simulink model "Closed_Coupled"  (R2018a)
settings: Solver=ode45  StartTime=0.0  StopTime=60  RelTol=1e-3  EnableMultiTasking=on
InitFcn:
  | init
StartFcn:
  | init
StopFcn:
  | pl
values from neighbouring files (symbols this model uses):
  Aact = [0, 1; -omg^2, -2*zet*omg]    [init.m]
  Bact = [0; omg^2]    [init.m]
  Cact = [1, 0]    [init.m]
  Cyb = -0.0245    [init.m]    (also in lqr_des.m)
  Cydel = [-0.24668,0.24668, 0.47413,-0.47413,0]/100    [init.m]    (also in lqr_des.m = [-0.24668,0.24668, 0.47413,-0.47413]/100)
  Cza = -0.073    [init.m]
  Czdel = [0.51664,0.51664,0.60478,0.60478,0.06]/100    [init.m]
  d2r = pi/180    (= 0.0174532925199)    [init.m]
  Dact = 0    [init.m]
  Mass = 198.32    [init.m]    (also in lqr_des.m)
  Qbar = 150    [init.m]    (also in lqr_des.m)
  r2d = 180/pi    (= 57.2957795131)    [init.m]    (also in pl.m)
  Sref = 79.069    [init.m]    (also in lqr_des.m)
  V0 = 822.8    [init.m]
undefined symbols (not defined in the file or in its folder): Ap, Bp, Cp, Dp, K4axmix, Kpr, Kq

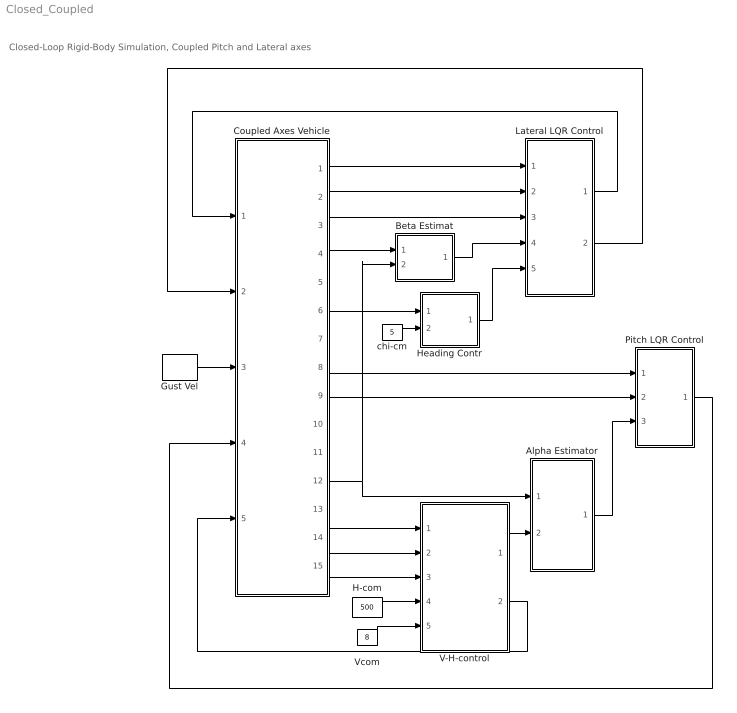
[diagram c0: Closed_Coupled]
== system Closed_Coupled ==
  note: Closed-Loop Rigid-Body Simulation, Coupled Pitch and Lateral axes
  Alpha Estimator : Subsystem
  Beta Estimat : Subsystem
  Coupled Axes Vehicle : Subsystem
  Gust Vel : DiscretePulseGenerator  PulseType=Time based  Amplitude=40  Period=100  PulseWidth=10  PhaseDelay=20
  H-com : Constant  Value=500
  Heading Contr : Subsystem
  Lateral LQR Control : Subsystem
  Pitch LQR Control : Subsystem
  V-H-control : Subsystem
  Vcom : Constant  Value=8
  chi-cm : Constant  Value=5
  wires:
  Coupled Axes Vehicle/2(p) -> Lateral LQR Control/2(p)
  Coupled Axes Vehicle/3(r) -> Lateral LQR Control/3(r)
  Coupled Axes Vehicle/1(phi) -> Lateral LQR Control/1(phi)
  Coupled Axes Vehicle/9(q) -> Pitch LQR Control/2(q)
  Coupled Axes Vehicle/8(thet) -> Pitch LQR Control/1(thet)
  Pitch LQR Control/1(elev) -> Coupled Axes Vehicle/4(pitch)
  Coupled Axes Vehicle/12(delt) -> Alpha Estimator/1(delta), Beta Estimat/2(delta)
  H-com/1 -> V-H-control/4(H-comd)
  Vcom/1 -> V-H-control/5(Vcomd)
  Alpha Estimator/1(alphat) -> Pitch LQR Control/3(alfa)
  V-H-control/1(Zdd-com) -> Alpha Estimator/2(Zdd)
  V-H-control/2(Throtle) -> Coupled Axes Vehicle/5(Ax-cmd)
  Lateral LQR Control/1(Ailer) -> Coupled Axes Vehicle/1(roll)
  Lateral LQR Control/2(Rud) -> Coupled Axes Vehicle/2(yaw)
  Coupled Axes Vehicle/4(Ny) -> Beta Estimat/1(Ydd)
  Beta Estimat/1(bethat) -> Lateral LQR Control/4(bet)
  chi-cm/1 -> Heading Contr/2(chi-cmd)
  Heading Contr/1(phi-cmd) -> Lateral LQR Control/5(ph-cmd)
  Coupled Axes Vehicle/6("chi ") -> Heading Contr/1(chi)
  Coupled Axes Vehicle/14(Nz) -> V-H-control/2(Az)
  Coupled Axes Vehicle/15(dH) -> V-H-control/3(dH)
  Coupled Axes Vehicle/13(V-dot) -> V-H-control/1(Vdot)
  Gust Vel/1 -> Coupled Axes Vehicle/3(Gust)

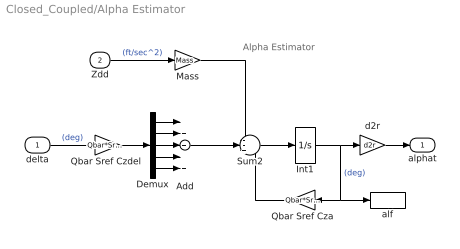
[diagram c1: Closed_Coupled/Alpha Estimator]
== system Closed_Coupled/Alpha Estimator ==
  note: Alpha Estimator
  delta : Inport
  Zdd : Inport  Port=2
  Add : Sum  Inputs=+++++
  Demux : Demux  Outputs=5
  Int1 : Integrator
  Mass : Gain  Gain=Mass
  Qbar Sref Cza : Gain  Gain=Qbar*Sref*Cza
  "Qbar Sref Czdel " : Gain  Gain=Qbar*Sref*Czdel
  Sum2 : Sum  Inputs=--+
  alf : ToWorkspace  VariableName=alphat  SampleTime=-1
  d2r : Gain  Gain=d2r
  alphat : Outport
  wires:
  Demux/5 -> Add/5
  Demux/4 -> Add/4
  Demux/3 -> Add/3
  Demux/2 -> Add/2
  Demux/1 -> Add/1
  "Qbar Sref Czdel "/1 -> Demux/1
  delta/1 -> "Qbar Sref Czdel "/1  "(deg)"
  Sum2/1 -> Int1/1
  Int1/1 -> d2r/1, Qbar Sref Cza/1, alf/1  "(deg)"
  Qbar Sref Cza/1 -> Sum2/3
  Zdd/1 -> Mass/1  "(ft/sec^2)"
  Mass/1 -> Sum2/1
  d2r/1 -> alphat/1
  Add/1 -> Sum2/2

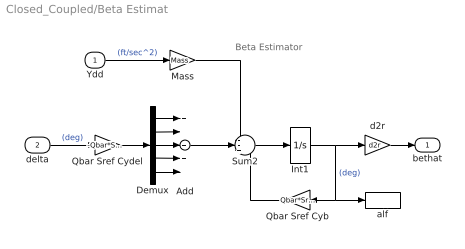
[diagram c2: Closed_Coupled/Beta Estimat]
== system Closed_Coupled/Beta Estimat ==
  note: Beta Estimator
  Ydd : Inport
  delta : Inport  Port=2
  Add : Sum  Inputs=+++++
  Demux : Demux  Outputs=5
  Int1 : Integrator
  Mass : Gain  Gain=Mass
  Qbar Sref Cyb : Gain  Gain=Qbar*Sref*Cyb
  Qbar Sref Cydel : Gain  Gain=-Qbar*Sref*Cydel
  Sum2 : Sum  Inputs=--+
  alf : ToWorkspace  VariableName=bethat  SampleTime=-1
  d2r : Gain  Gain=d2r
  bethat : Outport
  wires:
  Add/1 -> Sum2/2
  d2r/1 -> bethat/1
  Mass/1 -> Sum2/1
  Ydd/1 -> Mass/1  "(ft/sec^2)"
  Qbar Sref Cyb/1 -> Sum2/3
  Int1/1 -> alf/1, Qbar Sref Cyb/1, d2r/1  "(deg)"
  Sum2/1 -> Int1/1
  delta/1 -> Qbar Sref Cydel/1  "(deg)"
  Qbar Sref Cydel/1 -> Demux/1
  Demux/1 -> Add/1
  Demux/2 -> Add/2
  Demux/3 -> Add/3
  Demux/4 -> Add/4
  Demux/5 -> Add/5

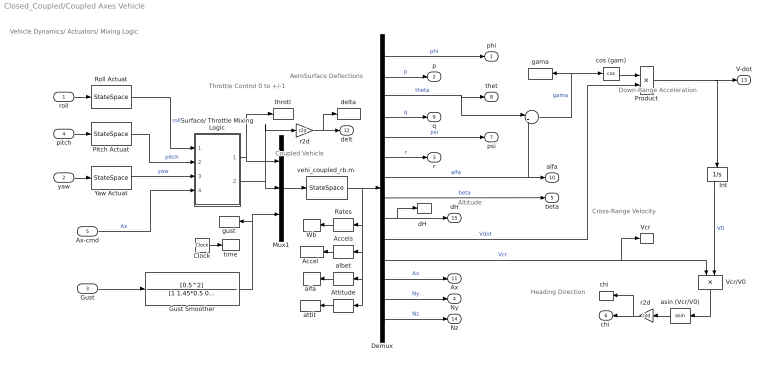
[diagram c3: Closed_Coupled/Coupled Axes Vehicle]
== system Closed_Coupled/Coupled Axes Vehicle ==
  note: Throttle Control 0 to +/-1
  note: Down-Range Acceleration
  note: Heading Direction
  note: Vehicle Dynamics/ Actuators/ Mixing Logic
  note: AeroSurface Deflections
  note: Coupled Vehicle
  note: Cross-Range Velocity
  note: Altitude
  roll : Inport
  yaw : Inport  Port=2
  Gust : Inport  Port=3
  pitch : Inport  Port=4
  Ax-cmd : Inport  Port=5
  "    " : Sum  Inputs=|+-
  "Accel " : ToWorkspace  VariableName=Accel  SampleTime=-1
  Accels : Selector  InputPortWidth=14  IndexOptions=Index vector (dialog)  Indices=[12:14]  OutputSizes=1
  Attitude : Selector  InputPortWidth=14  IndexOptions=Index vector (dialog)  Indices=[1,3,5]  OutputSizes=1
  Clock : Clock
  Demux : Demux  Outputs=14
  Gust Smoother : TransferFcn  Numerator=[0.5^2]  Denominator=[1 1.45*0.5 0.5^2]
  Int : Integrator  InitialCondition=V0
  Mux1 : Mux  Inputs=[1, 5, 1]
  Pitch Actuat : StateSpace  A=Aact  B=Bact  C=Cact  D=Dact  InitialCondition=0
  Product : Product
  Rates : Selector  InputPortWidth=14  IndexOptions=Index vector (dialog)  Indices=[2,4,6]  OutputSizes=1
  Roll Actuat : StateSpace  A=Aact  B=Bact  C=Cact  D=Dact  InitialCondition=0
  Surface/ Throttle Mixing Logic : Subsystem
  "Vcr " : ToWorkspace  VariableName=Vcr  SampleTime=-1
  Vcr/V0 : Product  Inputs=*/
  Wb : ToWorkspace  VariableName=Wb  SampleTime=-1
  Yaw Actuat : StateSpace  A=Aact  B=Bact  C=Cact  D=Dact  InitialCondition=0
  albet : Selector  InputPortWidth=14  IndexOptions=Index vector (dialog)  Indices=[7,8]  OutputSizes=1
  "alfa " : ToWorkspace  VariableName=alfa  SampleTime=-1
  asin (Vcr/V0) : Trigonometry  Operator=asin
  attit : ToWorkspace  VariableName=attit  SampleTime=-1
  "chi  " : ToWorkspace  VariableName=chi  SampleTime=-1
  cos (gam) : Trigonometry  Operator=cos
  "dH  " : ToWorkspace  VariableName=dH  SampleTime=-1
  delta : ToWorkspace  VariableName=delta  SampleTime=-1
  gama : ToWorkspace  VariableName=gama  SampleTime=-1
  gust : ToWorkspace  VariableName=gust  SampleTime=-1
  r2d : Gain  Gain=r2d
  "r2d " : Gain  Gain=r2d
  throtl : ToWorkspace  VariableName=Thro  SampleTime=-1
  time : ToWorkspace  VariableName=time  SampleTime=-1
  "vehi_coupled_rb.m " : StateSpace  A=Ap  B=Bp  C=Cp  D=Dp  InitialCondition=0
  phi : Outport
  p : Outport  Port=2
  r : Outport  Port=3
  Ny : Outport  Port=4
  beta : Outport  Port=5
  "chi " : Outport  Port=6
  psi : Outport  Port=7
  thet : Outport  Port=8
  q : Outport  Port=9
  alfa : Outport  Port=10
  Ax : Outport  Port=11
  delt : Outport  Port=12
  V-dot : Outport  Port=13
  Nz : Outport  Port=14
  dH : Outport  Port=15
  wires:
  Mux1/1 -> "vehi_coupled_rb.m "/1
  Gust/1 -> Gust Smoother/1
  Yaw Actuat/1 -> Surface/ Throttle Mixing Logic/3(yaw)  "yaw"
  Demux/1 -> phi/1  "phi"
  Demux/2 -> p/1  "p"
  roll/1 -> Roll Actuat/1
  yaw/1 -> Yaw Actuat/1
  pitch/1 -> Pitch Actuat/1
  Roll Actuat/1 -> Surface/ Throttle Mixing Logic/1(roll)  "roll"
  Pitch Actuat/1 -> Surface/ Throttle Mixing Logic/2(ptch)  "pitch"
  Ax-cmd/1 -> Surface/ Throttle Mixing Logic/4(Ax)  "Ax"
  "vehi_coupled_rb.m "/1 -> Demux/1, Attitude/1, albet/1, Accels/1, Rates/1
  Demux/3 -> thet/1, "    "/1  "theta"
  Demux/4 -> q/1  "q"
  Demux/5 -> psi/1  "psi"
  Demux/6 -> r/1  "r"
  Demux/7 -> alfa/1, "    "/2  "alfa"
  Demux/8 -> beta/1  "beta"
  Demux/9 -> dH/1, "dH  "/1
  Demux/11 -> Vcr/V0/1, "Vcr "/1  "Vcr"
  Demux/12 -> Ax/1  "Ax"
  Demux/13 -> Ny/1  "Ny"
  Demux/14 -> Nz/1  "Nz"
  r2d/1 -> delta/1, delt/1
  Gust Smoother/1 -> Mux1/3, gust/1
  Surface/ Throttle Mixing Logic/1(Thro) -> Mux1/1, throtl/1
  Surface/ Throttle Mixing Logic/2(delta) -> Mux1/2, r2d/1
  "    "/1 -> cos (gam)/1, gama/1  "gama"
  cos (gam)/1 -> Product/1
  Product/1 -> Int/1, V-dot/1
  Demux/10 -> Product/2  "Vdot"
  Int/1 -> Vcr/V0/2  "V0"
  "r2d "/1 -> "chi "/1, "chi  "/1
  Vcr/V0/1 -> asin (Vcr/V0)/1
  asin (Vcr/V0)/1 -> "r2d "/1
  Clock/1 -> time/1
  Rates/1 -> Wb/1
  Accels/1 -> "Accel "/1
  albet/1 -> "alfa "/1
  Attitude/1 -> attit/1

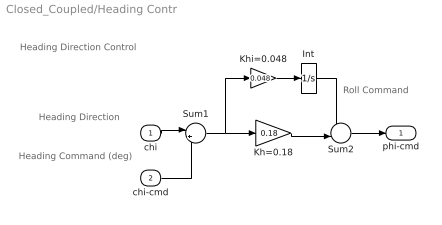
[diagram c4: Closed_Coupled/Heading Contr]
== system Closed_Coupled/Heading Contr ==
  note: Heading Direction Control
  note: Heading Direction
  note: Roll Command
  note: Heading Command (deg)
  chi : Inport
  chi-cmd : Inport  Port=2
  Int : Integrator
  Kh=0.18 : Gain  Gain=0.18
  Khi=0.048 : Gain  Gain=0.048
  Sum1 : Sum  Inputs=|+-
  Sum2 : Sum  Inputs=--|
  phi-cmd : Outport
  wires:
  Khi=0.048/1 -> Int/1
  Sum2/1 -> phi-cmd/1
  Sum1/1 -> Kh=0.18/1, Khi=0.048/1
  chi/1 -> Sum1/1
  chi-cmd/1 -> Sum1/2
  Kh=0.18/1 -> Sum2/2
  Int/1 -> Sum2/1

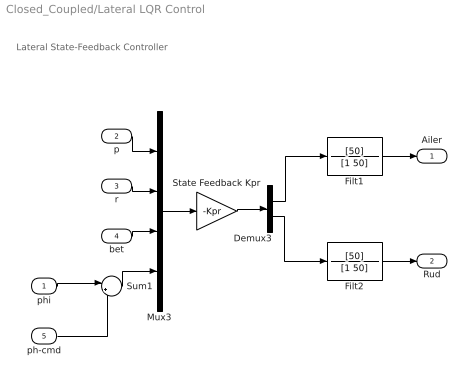
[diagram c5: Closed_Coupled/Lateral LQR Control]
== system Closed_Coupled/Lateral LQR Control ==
  note: Lateral State-Feedback Controller
  phi : Inport
  p : Inport  Port=2
  r : Inport  Port=3
  bet : Inport  Port=4
  ph-cmd : Inport  Port=5
  Demux3 : Demux  Outputs=2
  Filt1 : TransferFcn  Numerator=[50]  Denominator=[1 50]
  Filt2 : TransferFcn  Numerator=[50]  Denominator=[1 50]
  Mux3 : Mux
  State Feedback Kpr : Gain  Gain=-Kpr  Multiplication=Matrix(K*u) (u vector)
  Sum1 : Sum  Inputs=|+-
  Ailer : Outport
  Rud : Outport  Port=2
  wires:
  Mux3/1 -> State Feedback Kpr/1
  p/1 -> Mux3/1
  r/1 -> Mux3/2
  bet/1 -> Mux3/3
  Demux3/1 -> Filt1/1
  Demux3/2 -> Filt2/1
  Filt2/1 -> Rud/1
  Filt1/1 -> Ailer/1
  Sum1/1 -> Mux3/4
  phi/1 -> Sum1/1
  ph-cmd/1 -> Sum1/2
  State Feedback Kpr/1 -> Demux3/1

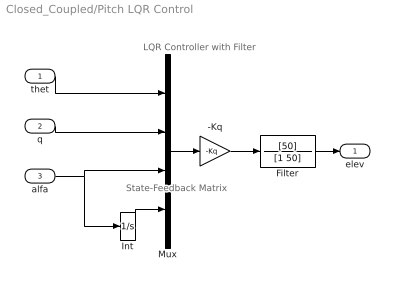
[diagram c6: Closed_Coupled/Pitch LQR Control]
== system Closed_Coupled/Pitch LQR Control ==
  note: LQR Controller with Filter
  note: State-Feedback Matrix
  thet : Inport
  q : Inport  Port=2
  alfa : Inport  Port=3
  -Kq : Gain  Gain=-Kq  Multiplication=Matrix(K*u)
  Filter : TransferFcn  Numerator=[50]  Denominator=[1 50]
  Int : Integrator
  Mux : Mux
  elev : Outport
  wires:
  -Kq/1 -> Filter/1
  Mux/1 -> -Kq/1
  Int/1 -> Mux/4
  Filter/1 -> elev/1
  q/1 -> Mux/2
  thet/1 -> Mux/1
  alfa/1 -> Mux/3, Int/1

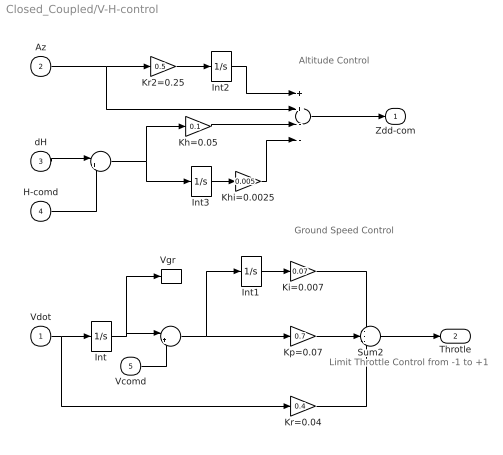
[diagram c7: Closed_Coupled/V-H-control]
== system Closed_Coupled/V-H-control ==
  note: Altitude Control
  note: Ground Speed Control
  note: Limit Throttle Control from -1 to +1
  Vdot : Inport
  Az : Inport  Port=2
  dH : Inport  Port=3
  H-comd : Inport  Port=4
  Vcomd : Inport  Port=5
  " " : Sum  Inputs=|+-
  "  " : Sum  Inputs=++--
  "    " : Sum  Inputs=|+-
  Int{,1..3} (4 alike) : Integrator
  Kh=0.05 : Gain  Gain=0.1
  Khi=0.0025 : Gain  Gain=0.005
  Ki=0.007 : Gain  Gain=0.07
  Kp=0.07 : Gain  Gain=0.7
  Kr2=0.25 : Gain  Gain=0.5
  Kr=0.04 : Gain  Gain=0.4
  Sum2 : Sum  Inputs=---
  "Vgr  " : ToWorkspace  VariableName=Vgr  SampleTime=-1
  Zdd-com : Outport
  Throtle : Outport  Port=2
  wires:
  Khi=0.0025/1 -> "  "/4
  Int3/1 -> Khi=0.0025/1
  " "/1 -> Int3/1, Kh=0.05/1
  "  "/1 -> Zdd-com/1
  Az/1 -> "  "/2, Kr2=0.25/1
  Int2/1 -> "  "/1
  Kr2=0.25/1 -> Int2/1
  Kh=0.05/1 -> "  "/3
  H-comd/1 -> " "/2
  dH/1 -> " "/1
  Vcomd/1 -> "    "/2
  "    "/1 -> Int1/1, Kp=0.07/1
  Int/1 -> "    "/1, "Vgr  "/1
  Int1/1 -> Ki=0.007/1
  Ki=0.007/1 -> Sum2/1
  Kp=0.07/1 -> Sum2/2
  Kr=0.04/1 -> Sum2/3
  Sum2/1 -> Throtle/1
  Vdot/1 -> Kr=0.04/1, Int/1

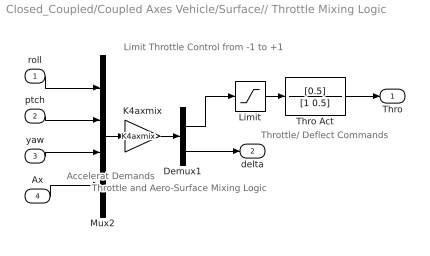
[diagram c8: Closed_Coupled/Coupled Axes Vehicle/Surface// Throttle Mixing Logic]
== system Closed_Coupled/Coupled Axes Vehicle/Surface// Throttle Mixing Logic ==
  note: Limit Throttle Control from -1 to +1
  note: Throttle and Aero-Surface Mixing Logic
  note: Accelerat Demands
  note: Throttle/ Deflect Commands
  roll : Inport
  ptch : Inport  Port=2
  yaw : Inport  Port=3
  Ax : Inport  Port=4
  Demux1 : Demux  Outputs=[1, 5]
  K4axmix : Gain  Gain=K4axmix  Multiplication=Matrix(K*u) (u vector)
  Limit : Saturate  UpperLimit=1  LowerLimit=-1
  Mux2 : Mux
  Thro Act : TransferFcn  Numerator=[0.5]  Denominator=[1 0.5]
  Thro : Outport
  delta : Outport  Port=2
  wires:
  Thro Act/1 -> Thro/1
  Limit/1 -> Thro Act/1
  K4axmix/1 -> Demux1/1
  Mux2/1 -> K4axmix/1
  Demux1/1 -> Limit/1
  Demux1/2 -> delta/1
  roll/1 -> Mux2/1
  Ax/1 -> Mux2/4
  yaw/1 -> Mux2/3
  ptch/1 -> Mux2/2
